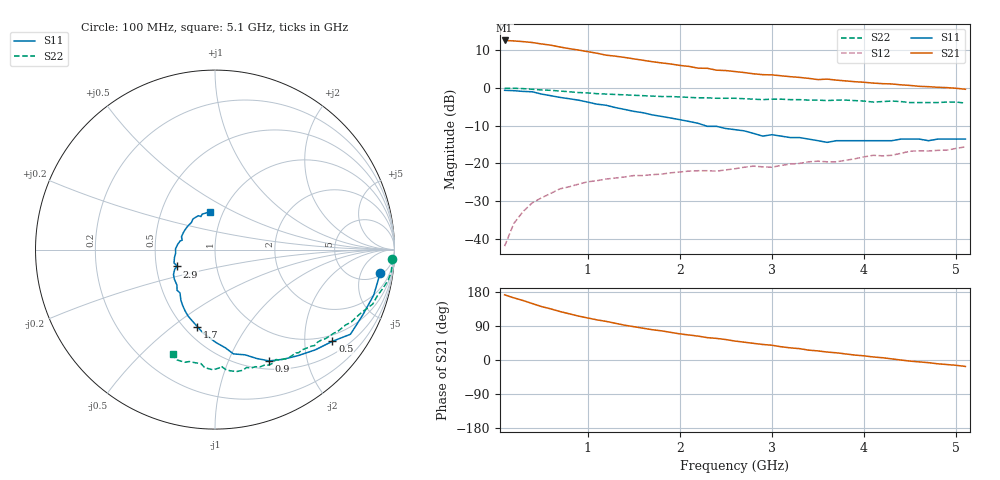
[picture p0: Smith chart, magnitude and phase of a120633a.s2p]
!  INA-12063 S PARAMETERS
!  Vd = 3 V  Id = 1.5 mA  LAST UPDATED 10-07-96
# ghz s ma r 50
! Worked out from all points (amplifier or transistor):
!   51 points, 100 MHz to 5.1 GHz, reference 50 ohm
!   highest |S21| = 12.6 dB at 100 MHz (marker M1)
!   |S21| within 3 dB of that: start of sweep to 1.01 GHz
!   unconditionally stable (mu >= 1): 1.515 GHz to end of sweep
!   at 900 MHz: K = 0.61, MSG = 17.8 dB, |S12| = -25.5 dB
!   at 2.6 GHz: K = 1.57, MAG = 8.4 dB, |S12| = -21.4 dB
!   at 5.1 GHz: K = 1.76, MAG = 2.6 dB, |S12| = -15.6 dB
!   S11 on the Smith chart (normalised r, x): 100 MHz: 6, -11; 500 MHz: 0.82, -2.68; 900 MHz: 0.60, -1.42; 1.7 GHz: 0.58, -0.62; 2.9 GHz: 0.64, -0.13; 5.1 GHz: 0.87, +0.38
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0.1  0.93 -8.0  4.26 172.0  0.008 86.0  0.99 -3.0
0.2  0.92 -16.0  4.2 164.0  0.016 79.0  0.99 -7.0
0.3  0.9 -24.0  4.11 157.0  0.023 73.0  0.98 -10.0
0.4  0.89 -32.0  4 149.0  0.03 69.0  0.96 -13.0
0.5  0.83 -38.0  3.83 141.0  0.035 64.0  0.94 -16.0
0.6  0.79 -45.0  3.69 135.0  0.04 60.0  0.93 -19.0
0.7  0.75 -52.0  3.49 128.0  0.046 56.0  0.91 -21.0
0.9  0.69 -64.0  3.18 116.0  0.053 50.0  0.87 -26.0
1  0.65 -69.0  3.03 111.0  0.057 47.0  0.86 -28.0
1.4  0.52 -89.0  2.54 92.0  0.066 40.0  0.81 -35.0
1.7  0.44 -103.0  2.23 80.0  0.071 35.0  0.78 -40.0
1.8  0.42 -107.0  2.15 77.0  0.072 35.0  0.77 -42.0
2  0.38 -116.0  1.99 69.0  0.077 33.0  0.76 -45.0
2.3  0.31 -129.0  1.82 59.0  0.08 30.0  0.74 -51.0
2.4  0.31 -133.0  1.72 57.0  0.079 29.0  0.73 -52.0
2.6  0.28 -144.0  1.65 50.0  0.085 30.0  0.73 -56.0
2.9  0.23 -156.0  1.5 41.0  0.09 24.0  0.7 -61.0
3.2  0.22 -175.0  1.41 32.0  0.098 28.0  0.7 -67.0
3.5  0.2 166.0  1.29 24.0  0.107 24.0  0.69 -73.0
3.6  0.19 164.0  1.31 21.0  0.105 23.0  0.68 -75.0
4.3  0.2 131.0  1.13 3.0  0.128 22.0  0.67 -91.0
5.1  0.21 98.0  0.96 -17.0  0.166 14.0  0.63 -112.0
